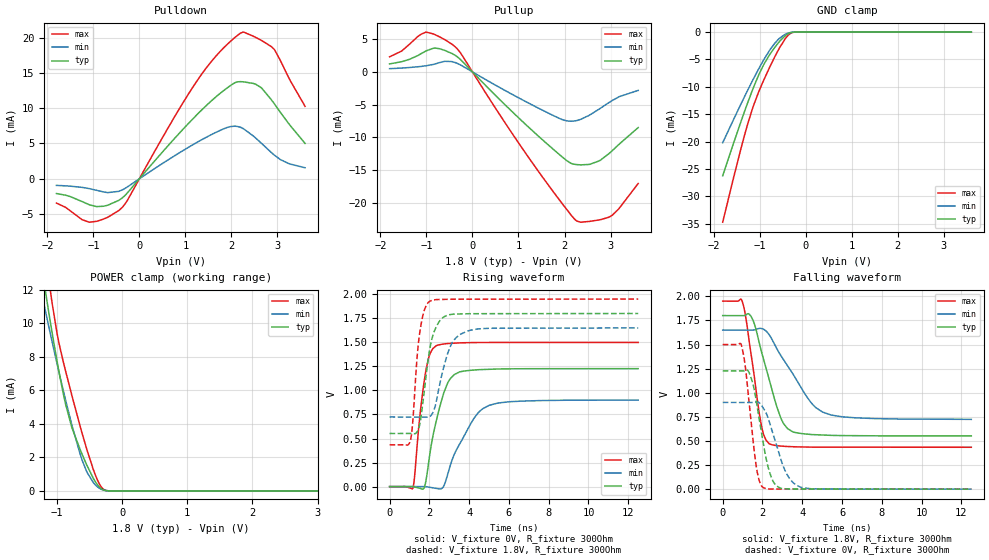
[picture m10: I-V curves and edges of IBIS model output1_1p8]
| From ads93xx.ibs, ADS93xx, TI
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|   output1_1p8 Model
[Model]   output1_1p8
Model_type   3-state
Polarity   Non-Inverting
Vmeas = 0.9
Vref = 0
Cref = 2pF
Rref = 100000
|   typ   min   max
C_comp   0.730pF   0.567pF   0.775pF
[Voltage Range]   1.8   1.65   1.95
[Temperature Range]   27   125   -40
[Pullup Reference]   1.8   1.65   1.95
[Pulldown Reference]   0   0   0
[Power Clamp Reference]   1.8   1.65   1.95
[GND Clamp Reference]   0   0   0
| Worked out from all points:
|   slope of the pulldown table from 0 to 0.27 V, typ, clamps not added: 131 ohm
|   slope of the pullup table from 0 to 0.27 V, typ, clamps not added: 138 ohm
|   GND clamp passes 1 mA (typ) near -0.48 V on its own axis
|   POWER clamp passes 1 mA (typ) near -0.47 V on its own axis
|   falling waveform, V_fixture 1.8V, R_fixture 300Ohm: 20-80 % time 1.01ns typ, 1.7ns min, 622ps max; typ from 1.8 V to 0.552 V
|   rising waveform, V_fixture 0V, R_fixture 300Ohm: 20-80 % time 777ps typ, 1.28ns min, 484ps max; typ from 0 V to 1.23 V
|   rising waveform, V_fixture 1.8V, R_fixture 300Ohm: 20-80 % time 517ps typ, 699ps min, 362ps max; typ from 0.552 V to 1.8 V
|   falling waveform, V_fixture 0V, R_fixture 300Ohm: 20-80 % time 629ps typ, 854ps min, 467ps max; typ from 1.23 V to 0 V
[Pulldown]
|   Voltage   I(typ)   I(min)   I(max)
-1.8V     -2.08mA    -931.7uA   -3.435mA
-1.093V   -3.656mA   -1.38mA    -6.135mA
-774mV    -3.878mA   -1.863mA   -5.683mA
-444.6mV  -3.043mA   -1.769mA   -4.49mA
-266.4mV  -2.039mA   -1.175mA   -3.112mA
689.4mV   5.163mA    2.949mA    7.932mA
1.294V    9.353mA    5.31mA     14.25mA
1.899V    12.82mA    7.245mA    18.96mA
2.207V    13.75mA    7.267mA    20.65mA
2.65V     12.89mA    5.044mA    19.6mA
2.93V     10.64mA    3.369mA    18.33mA
3.6V      5.012mA    1.565mA    10.25mA
[GND Clamp]
|   Voltage   I(typ)   I(min)   I(max)
-1.8V     -26.25mA   -20.21mA   -34.72mA
-1.568V   -20.38mA   -16.03mA   -26.71mA
-1.39V    -16.01mA   -12.89mA   -20.83mA
-1.26V    -12.96mA   -10.66mA   -16.87mA
-1.13V    -10.09mA   -8.505mA   -13.41mA
-919.8mV  -6.124mA   -5.225mA   -8.988mA
-763.2mV  -3.905mA   -3.105mA   -6.125mA
-558mV    -1.639mA   -1.074mA   -2.766mA
-444.6mV  -687.9uA   -414.5uA   -1.249mA
-347.4mV  -177.3uA   -111.8uA   -351.2uA
-207mV    -3.81uA    -5.113uA   -4.887uA
3.6V      0A         0A         0A
[Pullup]
|   Voltage   I(typ)   I(min)   I(max)
-1.8V     1.215mA    490.9uA    2.298mA
-1.368V   1.914mA    668uA      4.215mA
-1.006V   3.205mA    933.8uA    6.068mA
-806.4mV  3.634mA    1.221mA    5.651mA
-369mV    2.499mA    1.408mA    3.784mA
937.8mV   -6.569mA   -3.71mA    -10.17mA
1.818V    -12.17mA   -6.86mA    -18.85mA
2.126V    -13.88mA   -7.518mA   -21.67mA
2.266V    -14.13mA   -7.417mA   -22.73mA
2.758V    -13.55mA   -5.645mA   -22.56mA
3.028V    -12.07mA   -4.401mA   -21.9mA
3.6V      -8.489mA   -2.824mA   -17.01mA
[POWER Clamp]
|   Voltage   I(typ)   I(min)   I(max)
-1.8V     29.13mA    22.73mA    38.22mA
-1.217V   12.88mA    11.44mA    15.47mA
-1.13V    10.74mA    9.875mA    12.75mA
-1.087V   9.709mA    9.107mA    11.52mA
-968.4mV  7.078mA    7.058mA    8.793mA
-865.8mV  5.13mA     5.375mA    7.115mA
-774mV    3.808mA    3.958mA    5.725mA
-644.4mV  2.459mA    2.187mA    3.849mA
-541.8mV  1.531mA    1.127mA    2.464mA
-331.2mV  161.8uA    118.5uA    297.9uA
-142.2mV  415nA      1.1uA      356.8nA
3.6V      0A         0A         0A
[Ramp]
R_load = 300
|   typ   min   max
dV/dt_r   0.735831/7.77422e-10   0.539551/1.28136e-09   0.899493/4.84022e-10
dV/dt_f   0.748741/1.01053e-09   0.555656/1.70089e-09   0.909384/6.22214e-10
[Falling Waveform]
V_fixture = 1.8V
V_fixture_min = 1.65V
V_fixture_max = 1.95V
R_fixture = 300Ohm
C_fixture = 0F
|   Time   V(typ)   V(min)   V(max)
0s        1.8V       1.65V      1.95V
987.5ps   1.8V       1.65V      1.944V
1.465ns   1.777V     1.65V      1.345V
1.948ns   1.427V     1.666V     656.3mV
2.339ns   1.136V     1.6V       470.8mV
2.903ns   747.5mV    1.392V     447.4mV
3.248ns   630.2mV    1.283V     442.7mV
4.437ns   567.1mV    898.9mV    436.1mV
5.014ns   561.7mV    800.2mV    435.8mV
12.5ns    552.1mV    723.9mV    434.4mV
[Rising Waveform]
V_fixture = 0V
V_fixture_min = 0V
V_fixture_max = 0V
R_fixture = 300Ohm
C_fixture = 0F
|   Time   V(typ)   V(min)   V(max)
0s        146.8nV    16.93uV    -223.5nV
1.179ns   -439.5uV   158.6uV    -10.7mV
1.54ns    -18.61mV   202.1uV    767mV
1.833ns   66.86mV    -746.3uV   1.217V
2.339ns   674.8mV    -18.33mV   1.464V
2.724ns   973.7mV    5.918mV    1.483V
3.248ns   1.164V     332.5mV    1.492V
4.247ns   1.212V     711.5mV    1.498V
5.014ns   1.22V      845.6mV    1.498V
12.5ns    1.226V     899.3mV    1.499V
[Rising Waveform]
V_fixture = 1.8V
V_fixture_min = 1.65V
V_fixture_max = 1.95V
R_fixture = 300Ohm
C_fixture = 0F
|   Time   V(typ)   V(min)   V(max)
0s        552.1mV    723.9mV    434.4mV
1.057ns   552.3mV    722.9mV    487.8mV
1.164ns   551.8mV    722.7mV    669.9mV
1.487ns   619.2mV    722.4mV    1.556V
1.737ns   977.8mV    722.2mV    1.829V
2.047ns   1.461V     733.1mV    1.93V
2.469ns   1.708V     1.011V     1.945V
3.06ns    1.789V     1.46V      1.948V
3.907ns   1.797V     1.617V     1.949V
12.5ns    1.8V       1.65V      1.95V
[Falling Waveform]
|Gnd
V_fixture = 0V
V_fixture_min = 0V
V_fixture_max = 0V
R_fixture = 300Ohm
C_fixture = 0F
|   Time   V(typ)   V(min)   V(max)
0s        1.226V     899.2mV    1.499V
939ps     1.226V     899.1mV    1.494V
1.144ns   1.232V     899.1mV    1.259V
1.482ns   1.119V     899.3mV    594mV
1.737ns   851.1mV    904.4mV    174.2mV
2.047ns   469mV      838.3mV    15.74mV
2.588ns   62.91mV    534.8mV    984.8uV
3.201ns   3.174mV    165.1mV    923.9uV
3.907ns   1.117mV    21.59mV    853.6uV
12.5ns    330nV      15.88uV    -278.1nV
